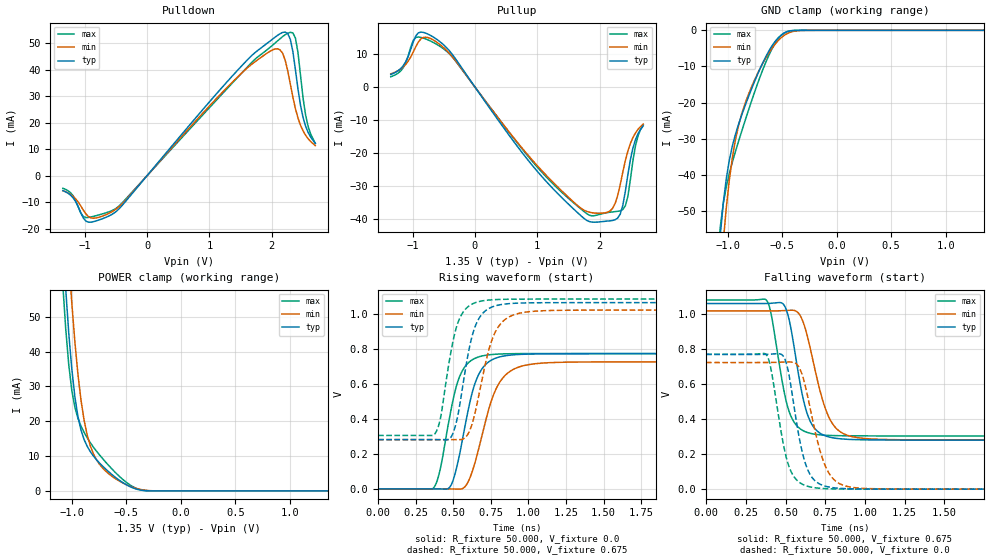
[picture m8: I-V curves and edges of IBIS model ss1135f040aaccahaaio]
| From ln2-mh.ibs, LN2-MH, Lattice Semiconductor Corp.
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|   Model ss1135f040aaccahaaio
[Model] ss1135f040aaccahaaio
| Clamp models do not include dynamic input termination. Please refer to
| the ss1135axxxaaccahaain model for input termination.
Model_type I/O
Polarity   Non-Inverting
Enable   Active-Low
Vinl =  0.575V
Vinh =  0.775V
Vmeas =  0.675V
Cref =  30.000pF
Rref =  50.000
Vref =  0.675V
C_comp   2.000pF   1.500pF   2.500pF
[Temperature Range]   25.000   0.125k   -40.000
[Voltage Range]   1.350V   1.310V   1.390V
[C Comp Corner]
C_comp   2.000pF   1.500pF   2.500pF
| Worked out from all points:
|   slope of the pulldown table from 0 to 0.203 V, typ, clamps not added: 35.6 ohm
|   slope of the pullup table from 0 to 0.203 V, typ, clamps not added: 36.9 ohm
|   GND clamp passes 1 mA (typ) near -0.50 V on its own axis
|   POWER clamp passes 1 mA (typ) near -0.45 V on its own axis
|   rising waveform, R_fixture 50.000, V_fixture 0.0: 20-80 % time 120ps typ, 148ps min, 109ps max; typ from 0 V to 0.771 V
|   rising waveform, R_fixture 50.000, V_fixture 0.675: 20-80 % time 103ps typ, 124ps min, 96.8ps max; typ from 0.281 V to 1.06 V
|   falling waveform, R_fixture 50.000, V_fixture 0.675: 20-80 % time 97.7ps typ, 126ps min, 93.1ps max; typ from 1.06 V to 0.281 V
|   falling waveform, R_fixture 50.000, V_fixture 0.0: 20-80 % time 93.7ps typ, 118ps min, 91.1ps max; typ from 0.771 V to 0 V
[Pulldown]
|Voltage   I(typ)   I(min)   I(max)
-1.35V    -5.611mA   -5.657mA   -4.743mA
-1.186V   -8.338mA   -7.786mA   -7.567mA
-981mV    -17.1mA    -14.39mA   -15.77mA
-530mV    -14.07mA   -13.09mA   -12.76mA
1.52V     41.41mA    38.71mA    38.69mA
2.012V    51.41mA    47.36mA    49.11mA
2.176V    53.96mA    46.1mA     52.41mA
2.299V    51.38mA    34.57mA    54.01mA
2.381V    39.95mA    25.26mA    51.84mA
2.463V    26.51mA    19.01mA    37.82mA
2.545V    18.62mA    15.22mA    22.77mA
2.7V      12.16mA    11.31mA    12.13mA
[Pullup]
|Voltage   I(typ)   I(min)   I(max)
-1.35V    3.79mA     3.988mA    3.105mA
-1.154V   6.383mA    6.037mA    5.758mA
-949mV    15.52mA    12.25mA    15.05mA
-826mV    16.57mA    15.06mA    14.83mA
-580mV    14.02mA    13.16mA    12.57mA
937mV     -24.15mA   -22.51mA   -22.91mA
1.839V    -40.83mA   -37.99mA   -38.92mA
2.208V    -40.48mA   -36.83mA   -37.88mA
2.331V    -38.55mA   -29.61mA   -37.54mA
2.413V    -31.67mA   -22.36mA   -36.05mA
2.536V    -18.44mA   -15.29mA   -22.19mA
2.7V      -11.83mA   -11.24mA   -11.45mA
[GND_clamp]
|Voltage   I(typ)   I(min)   I(max)
-1.35V    -224.6mA   -236.1mA   -220mA
-1.07V    -56.72mA   -69.44mA   -54.48mA
-1.042V   -47.78mA   -58.39mA   -47.95mA
-1.014V   -40.95mA   -48.99mA   -43.23mA
-986mV    -35.83mA   -41.27mA   -39.56mA
-930mV    -28.77mA   -30.24mA   -33.52mA
-846mV    -21.21mA   -20.61mA   -25.4mA
-734mV    -12.66mA   -12.39mA   -15.33mA
-622mV    -5.646mA   -6.175mA   -6.812mA
-482mV    -724.7uA   -1.376mA   -718.8uA
-314mV    -4.112uA   -39.82uA   -1.108uA
1.35V     0A         0A         0A
[POWER_clamp]
|Voltage   I(typ)   I(min)   I(max)
-1.338V   248.4mA    267.8mA    238.2mA
-1.086V   72.51mA    96.3mA     59.72mA
-1.058V   57.87mA    80.81mA    46.49mA
-1.03V    45.21mA    66.58mA    36.13mA
-1.002V   34.88mA    53.83mA    28.8mA
-946mV    21.35mA    33.5mA     20.88mA
-918mV    17.48mA    26.1mA     18.64mA
-862mV    12.87mA    16.19mA    15.31mA
-778mV    9.037mA    9.084mA    11.51mA
-610mV    4.102mA    3.705mA    5.539mA
-330mV    85.19uA    208uA      91.66uA
1.35V     0A         0A         0A
[Ramp]
| variable   typ   min   max
dV/dt_r   0.463/0.120n   0.435/0.148n   0.464/0.109n
dV/dt_f   0.472/0.107n   0.448/0.143n   0.469/96.233p
R_load = 50.000
[Rising Waveform]
R_fixture= 50.000
V_fixture= 0.0
V_fixture_min= 0.0
V_fixture_max= 0.0
|time   V(typ)   V(min)   V(max)
0s        1.215uV    6.808uV    559nV
368ps     66.39uV    48.23uV    4.991mV
475ps     8.607mV    -333.3uV   407.1mV
532ps     158.1mV    -1.293mV   617.9mV
604ps     469.7mV    49.89mV    722.5mV
667ps     649.5mV    222.8mV    752.7mV
758ps     736.7mV    514.5mV    766.8mV
894ps     764.5mV    679.3mV    771.4mV
1.208ns   770.9mV    722.2mV    772.4mV
10ns      771.2mV    725.1mV    772.5mV
[Rising Waveform]
R_fixture= 50.000
V_fixture= 0.675
V_fixture_min= 0.656
V_fixture_max= 0.696
|time   V(typ)   V(min)   V(max)
0s        280.9mV    281.2mV    304.7mV
375ps     280.9mV    281.2mV    311.6mV
416ps     280.4mV    281.2mV    410.7mV
483ps     293.5mV    280.8mV    776.4mV
537ps     449.6mV    281.1mV    962.6mV
612ps     825.4mV    338.7mV    1.048V
741ps     1.031V     807.5mV    1.078V
861ps     1.056V     976.3mV    1.082V
1.15ns    1.062V     1.018V     1.083V
10ns      1.063V     1.021V     1.083V
[Falling Waveform]
R_fixture= 50.000
V_fixture= 0.675
V_fixture_min= 0.656
V_fixture_max= 0.696
|time   V(typ)   V(min)   V(max)
0s        1.063V     1.02V      1.083V
379ps     1.063V     1.021V     1.083V
410ps     1.064V     1.021V     999.9mV
486ps     1.059V     1.022V     582.6mV
527ps     952.1mV    1.024V     433.8mV
605ps     542.8mV    970mV      338mV
723ps     317.3mV    543.5mV    310.6mV
833ps     289.5mV    336.5mV    306.2mV
1.084ns   281.7mV    285.6mV    304.9mV
10ns      280.9mV    281.2mV    304.7mV
[Falling Waveform]
R_fixture= 50.000
V_fixture= 0.0
V_fixture_min= 0.0
V_fixture_max= 0.0
|time   V(typ)   V(min)   V(max)
0s        771.2mV    725.1mV    772.5mV
379ps     771.8mV    725.2mV    770mV
484ps     763.6mV    727.4mV    269.4mV
521ps     657.9mV    728.4mV    132.1mV
595ps     255mV      678.8mV    34.25mV
649ps     93.24mV    489.7mV    14.17mV
713ps     30.51mV    233.6mV    5.438mV
813ps     7.079mV    48.02mV    1.43mV
1.029ns   663.8uV    3.036mV    163uV
10ns      1.198uV    6.785uV    544.5nV
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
